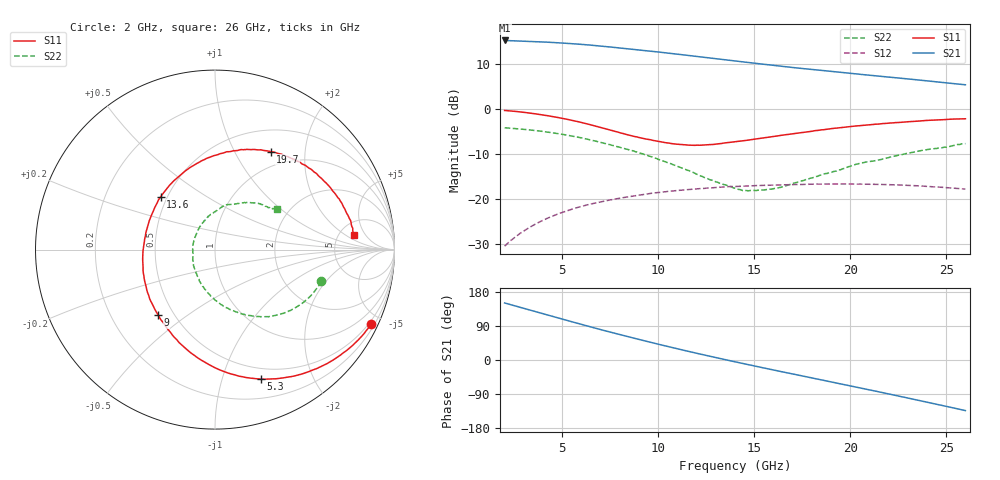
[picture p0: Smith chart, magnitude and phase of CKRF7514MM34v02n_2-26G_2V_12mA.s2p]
! CHUO DENSHI KOGYO Co.,Ltd.
! 22. July 2016
! CKRF7514MM34
! N-channel HJ-FET
! Vds = 2 V Id = 12 mA
# Hz S  MA  R 50
!	f	S11	S21	S12	S22
!	Hz	MAG	ANG	MAG	ANG	MAG	ANG	MAG	ANG
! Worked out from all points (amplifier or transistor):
!   241 points, 2 GHz to 26 GHz, reference 50 ohm
!   highest |S21| = 15.2 dB at 2 GHz (marker M1)
!   |S21| within 3 dB of that: start of sweep to 10.9 GHz
!   unconditionally stable (mu >= 1): 12.03 GHz to 19.12 GHz
!   at 6 GHz: K = 0.67, MSG = 18.0 dB, |S12| = -21.6 dB
!   at 14 GHz: K = 1.03, MAG = 12.9 dB, |S12| = -17.2 dB
!   at 26 GHz: K = 0.83, MSG = 11.6 dB, |S12| = -17.8 dB
!   lowest NFmin = 0.36 dB at 10 GHz
!   S11 on the Smith chart (normalised r, x): 2 GHz: 0.38, -4.37; 5.3 GHz: 0.39, -1.34; 9 GHz: 0.41, -0.39; 13.6 GHz: 0.46, +0.33; 19.7 GHz: 0.78, +1.41; 26 GHz: 6.79, +2.90
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2e9  0.9634 -25.6  5.767 150.5  0.03001 73.6  0.6186 -16.6
2.9e9  0.9242 -37.4  5.679 137.7  0.04289 66.8  0.5972 -24.1
3.7e9  0.8777 -48.2  5.59 126.3  0.05416 60.4  0.5732 -31.0
4.5e9  0.8246 -59.1  5.476 115.0  0.06475 54.4  0.5439 -37.8
5.3e9  0.7649 -70.5  5.347 103.7  0.07475 48.2  0.5107 -45.0
6e9  0.708 -80.8  5.219 94.0  0.08306 42.9  0.4788 -51.3
6.6e9  0.6578 -90.1  5.09 85.7  0.08908 38.3  0.4465 -56.6
7.4e9  0.5923 -102.9  4.904 74.9  0.09708 32.5  0.4052 -63.9
8.1e9  0.5386 -114.9  4.735 65.7  0.1029 27.7  0.3691 -70.5
9e9  0.4823 -131.1  4.526 54.3  0.1109 22.0  0.3272 -79.6
1e10  0.4365 -151.4  4.296 41.8  0.1182 15.0  0.2762 -90.9
1.08e10  0.4104 -168.2  4.108 32.0  0.1234 9.8  0.2398 -100.3
1.17e10  0.3965 172.7  3.901 21.3  0.1283 4.2  0.2018 -113.5
1.26e10  0.4007 154.1  3.703 11.0  0.1324 -1.4  0.1677 -129.0
1.36e10  0.4225 135.7  3.494 -0.3  0.1374 -7.9  0.1412 -150.5
1.4e10  0.4318 128.7  3.413 -4.8  0.1379 -10.4  0.132 -159.4
1.59e10  0.4916 101.5  3.072 -25.3  0.1431 -21.7  0.129 151.9
1.8e10  0.5661 77.2  2.751 -47.2  0.1464 -34.5  0.1715 109.3
1.97e10  0.6279 60.4  2.53 -65.1  0.1472 -45.4  0.2192 86.5
2.2e10  0.6973 40.1  2.262 -89.5  0.1446 -60.8  0.2885 62.8
2.39e10  0.7434 22.9  2.061 -110.4  0.1387 -75.2  0.3525 47.1
2.6e10  0.779 6.2  1.859 -133.6  0.129 -91.7  0.4124 33.4
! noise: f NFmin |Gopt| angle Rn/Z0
1e+10  0.36  0.427  102.4  0.06
1.05e+10  0.37  0.402  111.4  0.06
1.1e+10  0.38  0.37  121.1  0.05
1.15e+10  0.4  0.34  131.6  0.05
1.2e+10  0.43  0.313  144.1  0.04
1.25e+10  0.44  0.294  158  0.04
1.3e+10  0.46  0.281  171.9  0.04
1.35e+10  0.48  0.28  -172.9  0.04
1.4e+10  0.52  0.289  -158.2  0.04
1.5e+10  0.56  0.31  -135.4  0.05
